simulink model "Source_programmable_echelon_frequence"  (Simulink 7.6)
settings: Solver=ode23tb  StartTime=0.0  StopTime=0.2  RelTol=1e-3
PreLoadFcn:
  | delete *.mat
InitFcn:
  | T=1/60;
  | Arms=100;
StopFcn:
  | close all
  | load PhaseC.mat
  | plot(y(1,:),y(2,:))
  | grid
  | title('Tension phase C - Echelon de fréquence entre t=0.06s et t=0.14s')
  | axis([0 0.2 -6e-3 6e-3])
  | xlabel('temps')
  | 
  | figure
  | plot(y(1,:),y(3,:))
  | grid
  | title('Echelon de fréquence entre t=0.06s et t=0.14s')
  | ylabel('Amplitude tension phase C')
  | xlabel('temps')
  | 
  | delete *.mat
libraries: powerlib x6, powerlib_extras x1

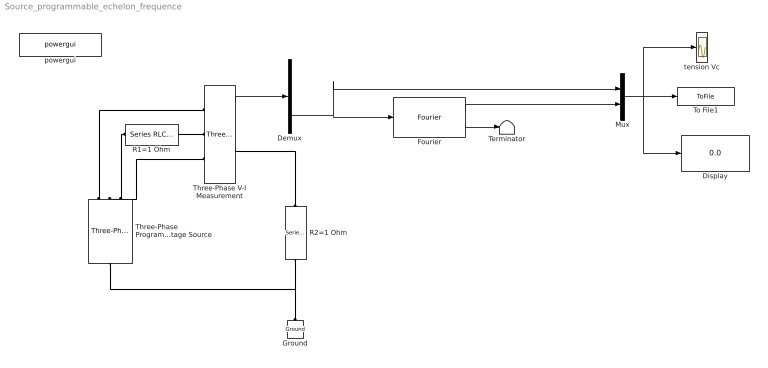
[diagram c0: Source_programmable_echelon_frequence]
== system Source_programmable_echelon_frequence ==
  Demux : Demux  Outputs=3
  Display : Display
  Fourier : powerlib_extras/Measurements/Fourier  DialogController=POWERSYS.PowerSysDialog  SystemSampleTime=-1  f1=60  n=2
  Ground : powerlib/Elements/Ground  DialogController=POWERSYS.PowerSysDialog  PhysicalDomain=powersysdomain  SubClassName=unknown  LeftPortType=p1  RightPortType=p1  LConnTagsString=a
  Mux : Mux  Inputs=2
  R1=1 Ohm : powerlib/Elements/Series RLC Branch  DialogController=POWERSYS.PowerSysDialog  PhysicalDomain=powersysdomain  SubClassName=unknown  LeftPortType=p1  RightPortType=p1  LConnTagsString=__new0  RConnTagsString=__new0  BranchType=R  Resistance=1  Inductance=1e-3  SetiL0=off  InitialCurrent=0  Capacitance=1e-6  Setx0=off  InitialVoltage=0  Measurements=None
  R2=1 Ohm : powerlib/Elements/Series RLC Branch  DialogController=POWERSYS.PowerSysDialog  PhysicalDomain=powersysdomain  SubClassName=unknown  LeftPortType=p1  RightPortType=p1  LConnTagsString=__new0  RConnTagsString=__new0  BranchType=R  Resistance=1  Inductance=1e-3  SetiL0=off  InitialCurrent=0  Capacitance=1e-6  Setx0=off  InitialVoltage=0  Measurements=None
  Terminator : Terminator
  Three-Phase Programmable Voltage Source : powerlib/Electrical Sources/Three-Phase Programmable Voltage Source  DialogController=POWERSYS.PowerSysDialog  SystemSampleTime=-1  PositiveSequence="[Arms  0 1/T]"  VariationEntity=Frequency  VariationType=Step  VariationStep=60  VariationRate=10  VariationMagnitude=0.3  VariationFrequency=2  VariationTiming="[0.06  0.14  0.2]"  VariationPhaseA=off  Amplitudes=[1 0.8 1.2 1.0]  TimeValues=[0 0.1 0.15 0.2]  HarmonicGeneration=off  HarmonicA="[3 0.2  -25 0]"  HarmonicB=[2 0.15 35 2]  Timing="[0.1  0.2]"
  Three-Phase V-I Measurement : powerlib/Measurements/Three-Phase V-I Measurement  DialogController=POWERSYS.PowerSysDialog  SystemSampleTime=-1  VoltageMeasurement=phase-to-ground  SetLabelV=off  LabelV=V1  Vpu=on  VpuLL=off  CurrentMeasurement=yes  SetLabelI=off  LabelI=I1  Ipu=on  Pbase=10e6  Vbase=25e3  OutputType=Magnitude  PhasorSimulation=off  PSBequivalent=0
  To File1 : ToFile  Filename=PhaseC  MatrixName=y
  powergui : powerlib/powergui  Priority=2  SystemSampleTime=-1  SimulationMode=Discrete  SampleTime=50e-6  frequency=60  SPID=off  DisableSnubberDevices=off  DisableRonSwitches=off  DisableVfSwitches=off  SwTol=0  Interpol=off  frequencyindice=60  echomessages=off  HookPort=off  DisplayEquations=off  FunctionMessages=off  EnableUseOfTLC=off  x0status=blocks  RestoreLinks=warning  ResistiveCurrentMeasurement=off  Frange=[0:2:500]  Ylog=off  Xlog=off  ShowGrid=off  save=off  variable=ZData  ZoomFFT=on  StartTime=0.0  cycles=1  DisplayStyle=off  fundamental=60  FreqAxis=off  MaxFrequency=1000  frequencyindicesteady=1  RmsSteady=1  display=off  Ts=0  methode=off
  tension Vc : Scope
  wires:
  Three-Phase V-I Measurement/1 -> Demux/1
  Demux/3 -> Fourier/1, Mux/1
  Fourier/1 -> Mux/2
  Fourier/2 -> Terminator/1
  Mux/1 -> To File1/1, tension Vc/1, Display/1
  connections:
  R2=1 Ohm/RConn1 -- Ground/LConn1 -- Three-Phase Programmable Voltage Source/LConn1
  R1=1 Ohm/LConn1 -- Three-Phase Programmable Voltage Source/RConn2
  R1=1 Ohm/RConn1 -- Three-Phase V-I Measurement/LConn2
  Three-Phase Programmable Voltage Source/RConn1 -- Three-Phase V-I Measurement/LConn1
  Three-Phase V-I Measurement/LConn3 -- Three-Phase Programmable Voltage Source/RConn3
  R2=1 Ohm/LConn1 -- Three-Phase V-I Measurement/RConn2
